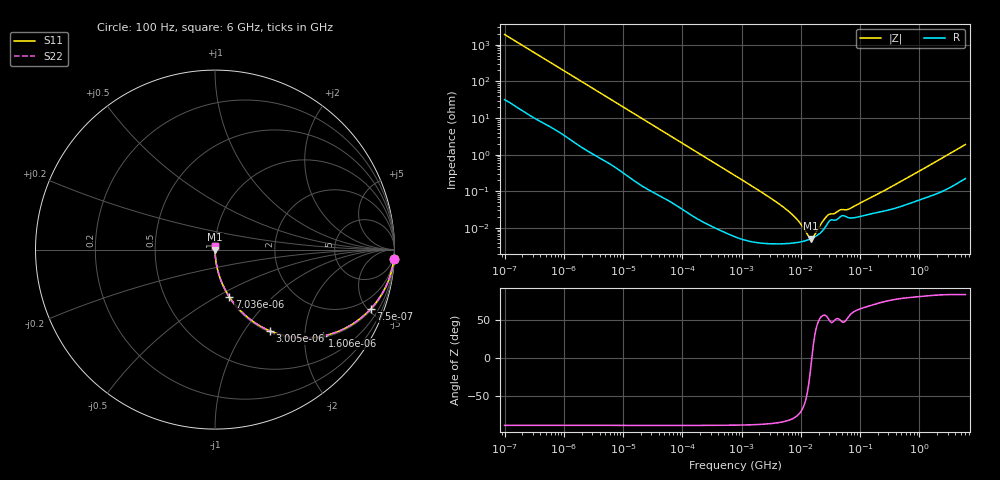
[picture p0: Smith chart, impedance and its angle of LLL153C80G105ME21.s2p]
!Murata Part Number: LLL153C80G105ME21
!These Parameters are Measured in Series Mode Connection
!Data Generated on Jan 08, 2026
!  o--ll--o
!Port1  Port2
!  o------o
!Operation Temp=25[degC], DC Bias Voltage=0[V]
!Freq. Start=100[Hz] Stop=6[GHz] 401[Steps]
# Hz S RI R 50
!Freq.(Hz) S11(Real) S11(Imag) S21(Real) S21(Imag) S12(Real) S12(Imag) S22(Real) S22(Imag)
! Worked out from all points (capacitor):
!   401 points, 100 Hz to 6 GHz, reference 50 ohm
!   read as one part in series: C = 828 nF near 109 Hz
!   lowest |Z| = 5.14 mohm at 14.88 MHz (marker M1)
!   series resonance near 15.33 MHz, so ESL is about 130 pH
!   S11 on the Smith chart (normalised r, x): 100 Hz: 2, -38; 750 Hz: 1.09, -5.22; 1.606 kHz: 1.04, -2.46; 3.005 kHz: 1.02, -1.32; 7.036 kHz: 1.01, -0.57; 6 GHz: 1.00, +0.04
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100  0.9964 -0.052  0.00358 0.052  0.00358 0.052  0.9964 -0.052
293  0.9754 -0.147  0.0246 0.147  0.0246 0.147  0.9754 -0.147
750  0.8678 -0.3301  0.1322 0.3301  0.1322 0.3301  0.8678 -0.3301
1606  0.6006 -0.4817  0.3994 0.4817  0.3994 0.4817  0.6006 -0.4817
2008  0.4929 -0.492  0.5071 0.492  0.5071 0.492  0.4929 -0.492
3005  0.307 -0.4533  0.693 0.4533  0.693 0.4533  0.307 -0.4533
4496  0.1686 -0.3662  0.8314 0.3662  0.8314 0.3662  0.1686 -0.3662
7036  0.0789 -0.2614  0.9211 0.2614  0.9211 0.2614  0.0789 -0.2614
15752  0.018 -0.1258  0.982 0.1258  0.982 0.1258  0.018 -0.1258
40335  0.00331 -0.0503  0.9967 0.0503  0.9967 0.0503  0.00331 -0.0503
774597  6.44e-05 -0.00269  0.9999 0.00269  0.9999 0.00269  6.44e-05 -0.00269
4856642  3.69e-05 -0.000389  1 0.000389  1 0.000389  3.69e-05 -0.000389
7266822  3.85e-05 -0.000225  1 0.000225  1 0.000225  3.85e-05 -0.000225
1.137099e7  4.37e-05 -8.36e-05  1 8.36e-05  1 8.36e-05  4.37e-05 -8.36e-05
1.487547e7  5.07e-05 -8.3e-06  0.9999 8.3e-06  0.9999 8.3e-06  5.07e-05 -8.3e-06
1.555665e7  5.24e-05 4.1e-06  0.9999 -4.1e-06  0.9999 -4.1e-06  5.24e-05 4.1e-06
1.946e7  6.46e-05 6.77e-05  0.9999 -6.77e-05  0.9999 -6.77e-05  6.46e-05 6.77e-05
3.045065e7  0.000156 0.00018  0.9998 -0.00018  0.9998 -0.00018  0.000156 0.00018
4.764863e7  0.000209 0.000237  0.9998 -0.000237  0.9998 -0.000237  0.000209 0.000237
6.817316e7  0.000187 0.000284  0.9998 -0.000284  0.9998 -0.000284  0.000187 0.000284
3.124326e8  0.000313 0.0012  0.9997 -0.0012  0.9997 -0.0012  0.000313 0.0012
6e9  0.00257 0.0187  0.9974 -0.0187  0.9974 -0.0187  0.00257 0.0187
